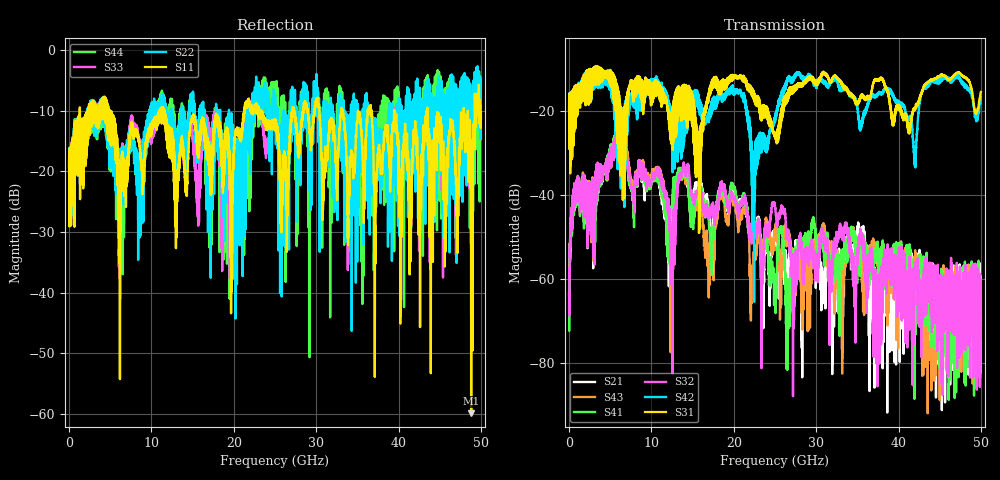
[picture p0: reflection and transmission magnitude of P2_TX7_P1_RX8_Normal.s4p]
!Keysight Technologies,N5225B,MY57041031,A.13.20.10
!Date: Friday, May 31, 2019 11:27:09
!Correction: S11(Full 4 Port(1,2,3,4))
!S12(Full 4 Port(1,2,3,4))
!S13(Full 4 Port(1,2,3,4))
!S14(Full 4 Port(1,2,3,4))
!S21(Full 4 Port(1,2,3,4))
!S22(Full 4 Port(1,2,3,4))
!S23(Full 4 Port(1,2,3,4))
!S24(Full 4 Port(1,2,3,4))
!S31(Full 4 Port(1,2,3,4))
!S32(Full 4 Port(1,2,3,4))
!S33(Full 4 Port(1,2,3,4))
!S34(Full 4 Port(1,2,3,4))
!S41(Full 4 Port(1,2,3,4))
!S42(Full 4 Port(1,2,3,4))
!S43(Full 4 Port(1,2,3,4))
!S44(Full 4 Port(1,2,3,4))
!S4P File: Measurements: <S11,S12,S13,S14>,
!<S21,S22,S23,S24>,
!<S31,S32,S33,S34>,
!<S41,S42,S43,S44>:
# Hz S  dB  R 50.0
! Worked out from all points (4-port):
!   5000 points, 10 MHz to 50 GHz, reference 50 ohm
!   strongest paths, dB at 10 MHz, 12.51 GHz, 25.01 GHz, 37.51 GHz, 50 GHz:
!     S31: -19.7, -21.0, -25.9, -12.8, -15.4
!     S42: -19.4, -24.4, -22.6, -15.9, -16.6
!     S32: -63.9, -52.2, -42.9, -68.3, -60.3
!     S41: -63.3, -42.3, -61.7, -54.9, -65.4
!     S43: -63.4, -50.6, -49.3, -56.0, -69.7
!     S21: -66.9, -45.2, -49.7, -70.3, -71.1
!   lowest |S11| = -59.9 dB at 48.82 GHz (marker M1), VSWR 1.00, Z = 50 + j0.0979 ohm
!   |S11| at or under -10 dB: 4.96 GHz to 10.98 GHz (6.02 GHz wide, 75.5 % of centre); 11.57 GHz to 21.26 GHz (9.683 GHz wide, 59 % of centre); 43.5 GHz to 47.91 GHz (4.407 GHz wide, 9.64 % of centre)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
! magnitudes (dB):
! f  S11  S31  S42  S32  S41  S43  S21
! 10 MHz  -20.2  -19.7  -19.4  -63.9  -63.3  -63.4  -66.9
! 6.24 GHz  -28.0  -18.9  -34.7  -25.8  -25.3  -25.5  -25.5
! 22.38 GHz  -10.3  -15.1  -39.9  -48.5  -47.7  -54.7  -47.5
! 26.56 GHz  -24.7  -16.3  -12.4  -48.4  -61.8  -51.5  -69.0
! 29.62 GHz  -13.0  -12.1  -12.8  -53.1  -45.3  -52.4  -53.5
! 48.82 GHz  -59.9  -14.2  -15.4  -69.0  -61.3  -67.7  -66.5
! 50 GHz  -11.2  -15.4  -16.6  -60.3  -65.4  -69.7  -71.1
